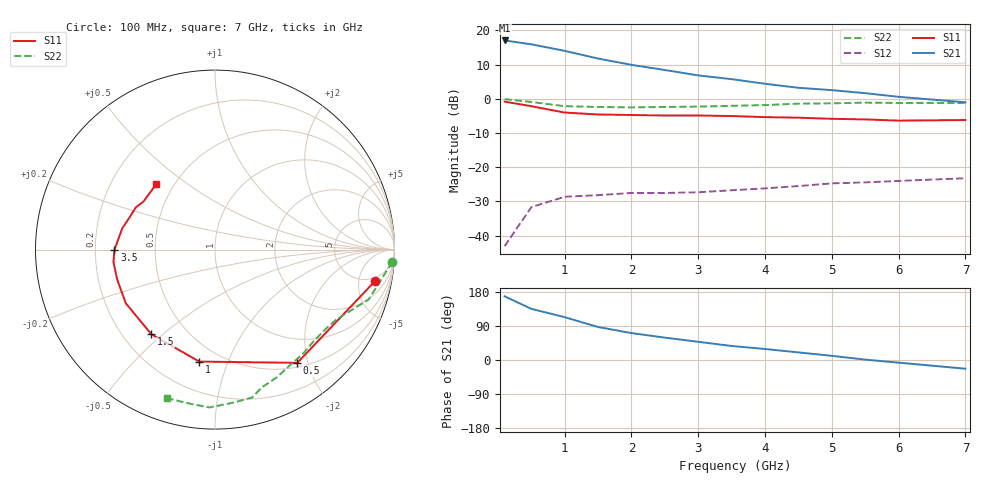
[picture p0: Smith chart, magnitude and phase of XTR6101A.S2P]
! HXTR-6101 (2N6617) Common Emitter
! Vce=10V  Ic=4mA
# ghz s ma r 50
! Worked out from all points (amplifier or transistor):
!   14 points, 100 MHz to 7 GHz, reference 50 ohm
!   highest |S21| = 17.1 dB at 100 MHz (marker M1)
!   |S21| within 3 dB of that: start of sweep to 988.9 MHz
!   unconditionally stable (mu >= 1): 1.882 GHz to 4.695 GHz; 5.841 GHz to end of sweep
!   at 1 GHz: K = 0.69, MSG = 21.3 dB, |S12| = -28.6 dB
!   at 3.5 GHz: K = 1.23, MAG = 13.4 dB, |S12| = -26.7 dB
!   at 7 GHz: K = 1.17, MAG = 8.6 dB, |S12| = -23.2 dB
!   S11 on the Smith chart (normalised r, x): 100 MHz: 4.14, -8.36; 500 MHz: 0.57, -1.83; 1 GHz: 0.38, -0.79; 1.5 GHz: 0.32, -0.46; 3.5 GHz: 0.28, +0.00; 7 GHz: 0.40, +0.38
0.1  0.91 -11.0  7.14 168.0  0.007 79.0  0.99 -4.0
0.5  0.78 -54.0  6.27 135.0  0.026 54.0  0.9 -18.0
1  0.63 -98.0  5.03 113.0  0.037 33.0  0.78 -30.0
1.5  0.59 -127.0  3.88 87.0  0.039 28.0  0.76 -35.0
2  0.58 -149.0  3.14 71.0  0.042 26.0  0.75 -43.0
2.5  0.57 -163.0  2.64 59.0  0.042 25.0  0.76 -50.0
3  0.57 -173.0  2.2 48.0  0.043 25.0  0.77 -58.0
3.5  0.56 180.0  1.94 37.0  0.046 25.0  0.79 -64.0
4  0.54 173.0  1.66 29.0  0.049 24.0  0.81 -71.0
4.5  0.53 167.0  1.45 20.0  0.053 24.0  0.85 -76.0
5  0.51 160.0  1.34 11.0  0.058 23.0  0.86 -84.0
5.5  0.5 152.0  1.21 1.0  0.06 22.0  0.88 -92.0
6  0.48 146.0  1.07 -7.0  0.063 20.0  0.87 -99.0
7  0.49 132.0  0.89 -23.0  0.069 15.0  0.87 -108.0
